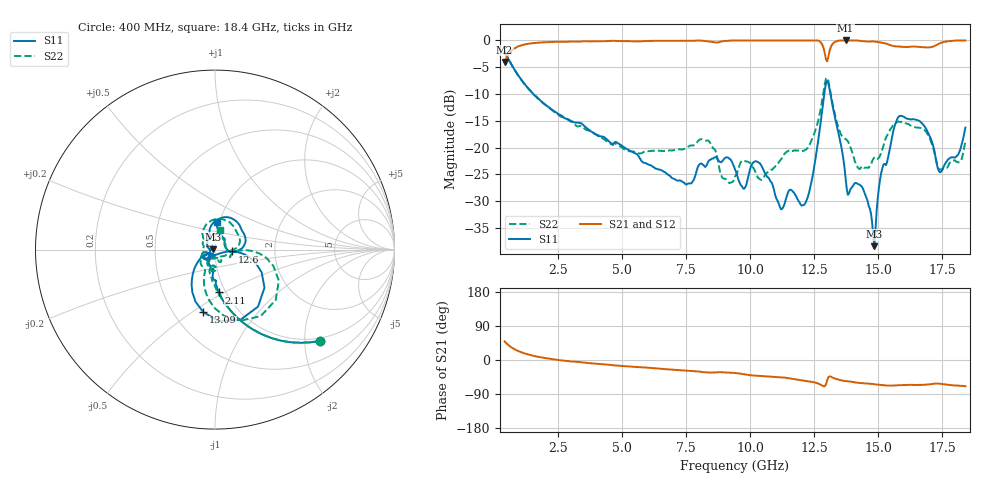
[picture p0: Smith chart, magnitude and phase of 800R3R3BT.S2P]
!  American Technical Ceramics  Date:  6/19/09
!  One Norden Lane
!  Huntington Station,  NY.  11746-2102
!  Tel:  (631) 622-4700  Fax:  (631) 622-4748
!  Part Number  800R3R3BT
!  Description: Ultra-low ESR, NPO  Mounting Orientation: Vertical
!  Application: High RF power Filters, Combiners, Matching networks,
!  Antenna, DC block, Bypass and Couplers
# GHZ S DB R 50
! Freq  |S11|  S11 Ph  |S21|  S21 Ph  |S12|  S12 Ph  |S22|  S22 Ph
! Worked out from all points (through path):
!   401 points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, 400 MHz to 18.4 GHz, reference 50 ohm
!   highest |S21| = 0.00 dB at 13.72 GHz (marker M1); lowest = -4.0 dB at 400 MHz (marker M2)
!   group delay of S21, straight-line fit = 14.1 ps
!   lowest |S11| = -38.4 dB at 14.85 GHz (marker M3), VSWR 1.02, Z = 48.8 + j0.176 ohm
!   |S11| at or under -10 dB: 1.525 GHz to 12.89 GHz (11.36 GHz wide, 158 % of centre); 13.13 GHz to end of sweep
!   |S22| runs from -26.6 to -2.2 dB; largest |S21 - S12| = 0.0048
!   S11 on the Smith chart (normalised r, x): 400 MHz: 0.93, -2.37; 2.11 GHz: 0.93, -0.47; 12.6 GHz: 1.21, -0.03; 13.09 GHz: 0.70, -0.56; 18.4 GHz: 0.97, +0.30
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0.4  -2.20 -40.9  -4.03 49.0  -4.06 49.0  -2.20 -40.9
1.03  -7.18 -68.8  -0.94 20.9  -0.96 20.9  -7.22 -68.9
2.11  -12.40 -84.9  -0.30 3.8  -0.31 3.8  -12.49 -86.5
3.415  -15.53 -92.3  -0.17 -6.0  -0.19 -5.9  -16.03 -97.2
6.43  -24.09 -123.7  -0.06 -22.7  -0.06 -22.6  -20.58 -93.1
8.32  -23.02 -130.5  -0.15 -32.8  -0.14 -32.6  -18.67 -101.9
9.4  -24.07 -165.7  -0.01 -34.3  -0.01 -34.2  -25.43 -64.8
9.76  -27.67 -140.9  -0.01 -37.8  -0.01 -37.6  -22.53 -67.6
10.345  -22.85 -144.3  -0.01 -41.9  -0.01 -41.8  -25.79 -60.8
11.2  -31.53 -122.5  -0.01 -45.6  -0.01 -45.5  -22.19 -23.3
12.415  -25.74 -16.9  -0.01 -57.8  -0.01 -57.8  -18.35 -4.5
12.595  -20.48 -6.2  -0.01 -61.0  -0.01 -61.0  -15.96 -1.4
12.91  -9.17 -37.6  -2.45 -69.1  -2.44 -69.2  -8.06 -25.9
13.09  -8.99 -100.5  -2.05 -43.1  -2.05 -43.1  -8.58 -82.3
13.72  -25.60 -150.7  0.00 -55.6  -0.01 -55.6  -18.38 -122.6
14.215  -26.82 -112.3  -0.04 -60.2  -0.03 -60.3  -23.83 -164.6
14.845  -38.40 171.4  -0.19 -64.0  -0.17 -64.1  -21.86 144.6
15.43  -20.59 109.0  -0.81 -67.8  -0.79 -67.8  -16.87 111.8
15.79  -14.22 68.3  -1.12 -66.5  -1.11 -66.7  -15.12 77.8
16.51  -14.85 20.8  -1.17 -66.0  -1.15 -66.2  -16.25 35.5
17.455  -24.48 27.2  -0.43 -63.1  -0.40 -63.2  -24.05 20.2
18.4  -16.27 86.9  -0.01 -69.4  -0.01 -69.6  -18.89 75.0
